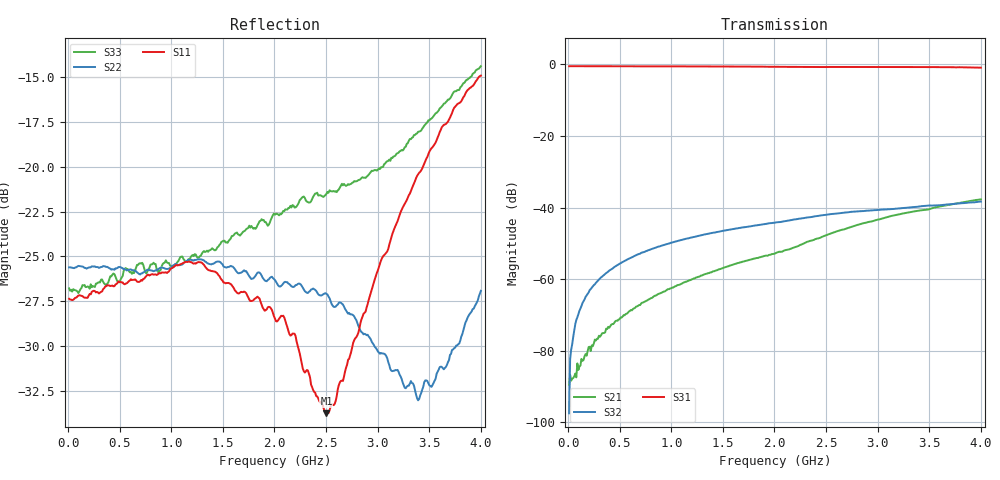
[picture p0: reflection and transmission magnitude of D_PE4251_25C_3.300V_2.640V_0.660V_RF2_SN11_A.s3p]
! Device ID: PE4251_SoldCshunt_081809
! Dir: c:\Test Bench Repositories\Bench_Software_CVI_Version_8\trunk\PSC 4Port_VNA Bench\datalog\4250\TEST\PE4251_SoldCshunt_081809\25C\3p300000\RF2
! Serial: 11
! Insertion: A
! Temp: 25C
! VDD: 3.300
! Control_Hi: 80.000
! Control_Lo: 20.000
! Logic State: RF2
! Port 1: RFC
! Port 2: RF1
! Port 3: RF2
! V1 = 0.66
! V2 = 0.66
! V3 = 0.66
! IDD: 4.662780e-05
! FILE NAME
! DATE 08/18/09  20:13
! CORRECTED  DATA
#  Hz  S  RI  R  50.00
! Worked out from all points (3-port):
!   401 points, 10 MHz to 4 GHz, reference 50 ohm
!   strongest paths, dB at 10 MHz, 1.008 GHz, 2.005 GHz, 3.002 GHz, 4 GHz:
!     S31: -0.6, -0.6, -0.7, -0.7, -1.0
!     S32: -97.5, -49.8, -44.2, -40.7, -38.3
!     S21: -89.5, -62.4, -52.8, -43.4, -37.7
!   lowest |S11| = -33.7 dB at 2.504 GHz (marker M1), VSWR 1.04, Z = 50.5 - j2 ohm
!   |S11| at or under -10 dB: start of sweep to end of sweep
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1e7  0.0429 -0.000604  -6.53e-06 -3.19e-05  0.9382 -0.00276
     2.03e-05 -2.68e-05  0.0524 -0.00093  1.42e-05 2.93e-05
     0.9379 -0.00415  1.34e-05 6.25e-07  0.0458 0.000319
3.9925e7  0.0425 0.00028  2.47e-05 -3.54e-05  0.939 -0.0157
          3.28e-05 -2.41e-05  0.0523 -0.000816  4.43e-05 0.000122
          0.9396 -0.0153  4.88e-05 0.000113  0.0449 5.78e-05
8.98e7  0.0435 0.00118  1.83e-05 -4.62e-05  0.9386 -0.0324
        2.08e-05 -6.33e-05  0.0527 -0.00112  3.86e-05 0.000285
        0.9395 -0.0324  4.36e-05 0.00029  0.0449 -0.000682
1.8955e8  0.0431 0.00219  -1.06e-05 -9.04e-05  0.9363 -0.0669
          8.71e-07 -9.9e-05  0.0522 -0.00161  5.65e-05 0.00062
          0.9362 -0.0664  6.41e-05 0.000623  0.0464 1.13e-05
4.98775e8  0.0477 0.00164  -0.000163 -0.000228  0.9202 -0.1712
           -0.000165 -0.00022  0.0524 -0.00432  0.000159 0.00163
           0.9205 -0.1718  0.000165 0.00163  0.0475 -0.00351
1.117225e9  0.0528 -0.0112  -0.000826 -0.000324  0.8566 -0.37
            -0.000832 -0.000326  0.0524 -0.0122  0.000546 0.00353
            0.8581 -0.3699  0.000541 0.00354  0.054 -0.0121
2.005e9  0.0351 -0.0138  -0.00223 -0.000409  0.6958 -0.6036
         -0.00224 -0.000411  0.0478 -0.00679  0.00117 0.00604
         0.6977 -0.6042  0.00116 0.00606  0.0663 -0.0317
2.50375e9  0.00565 -0.0198  -0.00403 -0.000843  0.5848 -0.7023
           -0.00403 -0.000847  0.0443 0.000152  0.0016 0.00776
           0.5872 -0.7025  0.0016 0.00775  0.0529 -0.0654
3.391525e9  -0.0872 -0.0383  -0.00899 0.00101  0.3466 -0.8449
            -0.00898 0.00102  0.0129 0.0183  0.00231 0.01
            0.3485 -0.8454  0.00229 0.01  -0.0274 -0.122
4e9  -0.1774 -0.0268  -0.0125 0.00365  0.1309 -0.8878
     -0.0125 0.00363  -0.0264 0.0366  0.00248 0.0118
     0.1321 -0.8864  0.00247 0.0119  -0.1342 -0.1353
